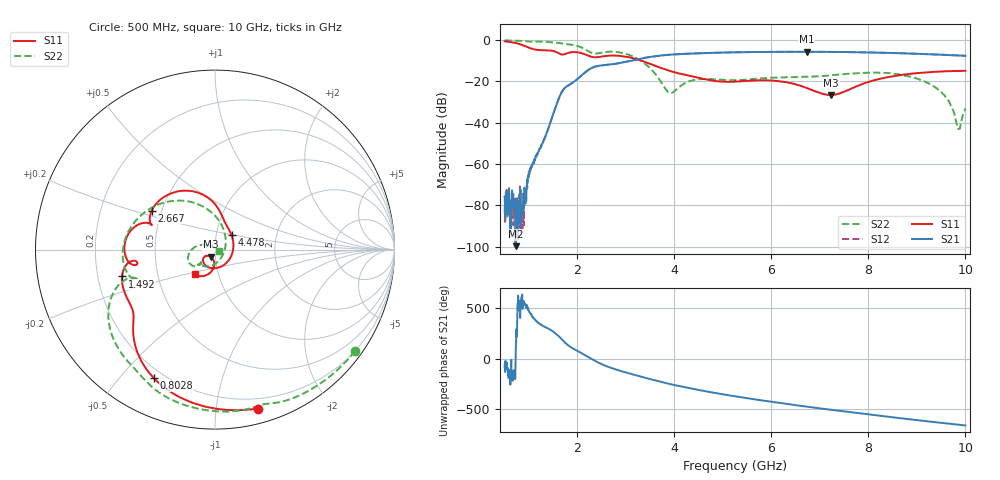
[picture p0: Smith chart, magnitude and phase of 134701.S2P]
!  2-Port S-parameters saved by WinCal
! VAR MeasName=S-Parameters (CALIBRATED_DATA) read from VNA (N5242A)
! VAR MeasDate=2013-7-3 16:18:31
! VAR NAME=134701
! VAR FILENAME=134701.S2P
! VAR DATE=2013-7-3 16:18:31
! VAR PHYS_PORTS=1,2
# Hz S MA R 50
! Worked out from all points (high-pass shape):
!   1601 points, 500 MHz to 10 GHz, reference 50 ohm
!   highest |S21| = -5.79 dB at 6.728 GHz (marker M1); lowest = -99.7 dB at 725.6 MHz (marker M2)
!   |S21| within 3 dB of the highest: 3.371 GHz to end of sweep
!   lowest |S11| = -26.7 dB at 7.233 GHz (marker M3), VSWR 1.10, Z = 47.5 - j3.76 ohm
!   |S11| at or under -10 dB: 3.31 GHz to end of sweep
!   |S22| runs from -43.1 to -0.3 dB; largest |S21 - S12| = 0.0028
!   S11 on the Smith chart (normalised r, x): 500 MHz: 0.12, -1.30; 802.8 MHz: 0.16, -0.62; 1.492 GHz: 0.31, -0.13; 2.667 GHz: 0.44, +0.23; 4.478 GHz: 1.19, +0.19; 10 GHz: 0.77, -0.22
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5e8  0.9173 -74.8  0.000164 -87.3  6.591e-05 -82.6  0.9627 -35.9
7.25625e8  0.8375 -105.6  1.041e-05 -56.3  0.0001328 -179.8  0.9488 -51.9
8.028125e8  0.7926 -115.5  3.669e-05 114.8  0.0001459 -164.6  0.9421 -57.5
8.978125e8  0.723 -126.3  0.0001906 -147.8  3.33e-05 116.1  0.9305 -64.3
1.0225e9  0.6297 -136.4  0.000782 98.9  0.0006959 94.2  0.9033 -72.4
1.491562e9  0.5388 -163.9  0.01481 -88.4  0.01489 -89.3  0.87 -106.3
1.705312e9  0.4392 -169.9  0.06149 178.1  0.06131 178.0  0.8072 -122.3
2.085312e9  0.4751 165.9  0.1379 54.0  0.1371 53.9  0.6532 -153.7
2.667188e9  0.4138 148.3  0.253 -87.9  0.2522 -87.9  0.5151 -171.7
3.195625e9  0.3471 110.8  0.3297 -164.5  0.3292 -164.3  0.3717 133.9
3.670625e9  0.2202 83.8  0.4114 134.6  0.411 134.7  0.119 65.5
3.92e9  0.1749 74.3  0.4375 105.6  0.4374 105.6  0.05186 -21.2
4.478125e9  0.1219 40.7  0.4703 49.5  0.4706 49.6  0.1104 -123.2
5.25e9  0.09747 -49.4  0.4985 -15.3  0.4988 -15.3  0.1058 -137.3
6.004062e9  0.1041 -117.6  0.5098 -70.2  0.5096 -70.3  0.1214 -136.2
6.728438e9  0.06872 -146.2  0.5135 -118.3  0.5123 -118.3  0.1277 -138.6
6.835312e9  0.0612 -145.1  0.5127 -125.1  0.5124 -125.1  0.1288 -138.4
7.233125e9  0.04616 -121.3  0.51 -149.8  0.5092 -149.9  0.1391 -138.7
8.420625e9  0.1268 -100.4  0.4813 140.0  0.4809 140.0  0.1571 -164.2
9.435938e9  0.1702 -119.6  0.438 84.1  0.4402 84.1  0.06344 154.4
9.8575e9  0.177 -126.8  0.4174 62.1  0.4189 62.0  0.007025 62.4
1e10  0.1779 -129.1  0.4107 54.6  0.4115 54.6  0.02202 -21.5
